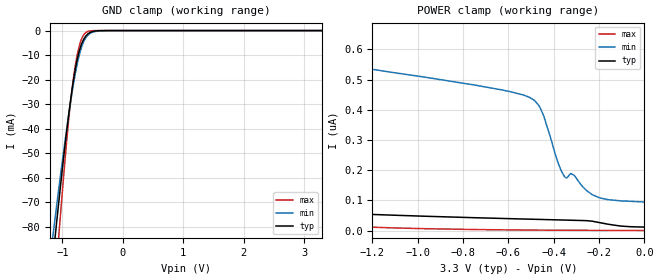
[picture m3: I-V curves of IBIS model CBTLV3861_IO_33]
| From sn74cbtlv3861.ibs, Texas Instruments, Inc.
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[Model]   CBTLV3861_IO_33
Model_type  Terminator
| variable   typ   min   max
C_comp   3.92pF   3.44pF   4.46pF
| C_tri-state   3.92pF   3.44pF   4.46pF
[Temperature Range]   40   100   -40
| Ambient temperature   25   85   -40
[Voltage range]   3.3   3   3.6
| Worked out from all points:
|   GND clamp passes 1 mA (typ) near -0.56 V on its own axis
[GND Clamp]
| CBTLV3861_IO_33
|   Voltage   I(typ)   I(min)   I(max)
-3.3V     -702.6mA   -588.6mA   -870mA
-1.17V    -96.27mA   -86.53mA   -119.2mA
-1.135V   -87.81mA   -79.47mA   -107.9mA
-1.1V     -79.47mA   -72.5mA    -96.72mA
-1.065V   -71.26mA   -65.63mA   -85.68mA
-1.035V   -64.36mA   -59.83mA   -76.37mA
-885mV    -32.39mA   -32.65mA   -33.92mA
-805mV    -18.56mA   -20.26mA   -17.42mA
-705mV    -7.13mA    -8.653mA   -5.017mA
-585mV    -1.526mA   -2.07mA    -421.5uA
-335mV    -12.16uA   -78.32uA   -273.3nA
3.3V      11.77nA    173.3nA    114.7pA
[POWER Clamp]
| CBTLV3861_IO_33
|   Voltage   I(typ)   I(min)   I(max)
-3.3V     168.9nA    755nA      3.102uA
-2.745V   120.8nA    701.8nA    664.5nA
-2.59V    110.6nA    686.5nA    444.6nA
-2.395V   99.23nA    667nA      273.1nA
-2.165V   87.67nA    643.5nA    157nA
-1.85V    74.37nA    609.9nA    63.84nA
-530mV    38.47nA    448.2nA    2.044nA
-460mV    37.11nA    406.8nA    1.706nA
-350mV    35nA       177.2nA    1.297nA
-310mV    34.23nA    183.3nA    1.176nA
-200mV    26.93nA    109.2nA    906.8pA
-48.03fV  11.77nA    94.8nA     587.4pA
